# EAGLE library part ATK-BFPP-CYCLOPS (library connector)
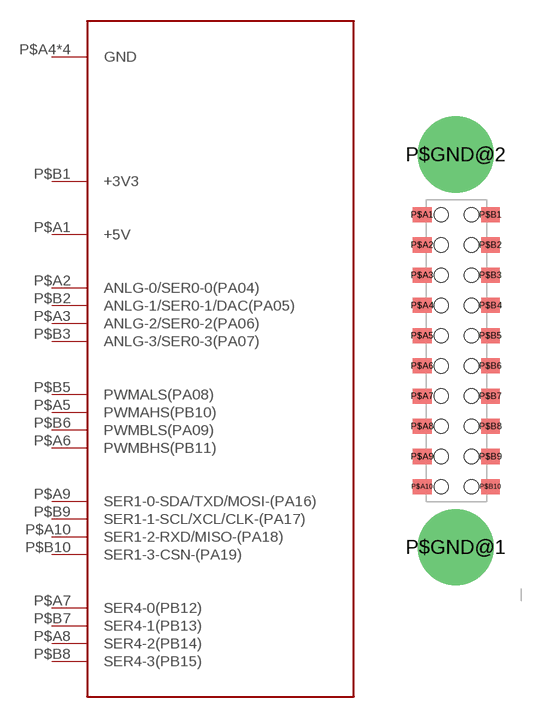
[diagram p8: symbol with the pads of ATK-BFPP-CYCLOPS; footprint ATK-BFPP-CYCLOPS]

Designator prefix J

## ATK-BFPP-CYCLOPSCYCLOPS  [ATK-BFPP-CYCLOPS]
P$A1  +5V
P$A2  ANLG-0/SER0-0(PA04)
P$A3  ANLG-2/SER0-2(PA06)
P$A4  GND
P$A5  PWMAHS(PB10)
P$A6  PWMBHS(PB11)
P$A7  SER4-0(PB12)
P$A8  SER4-2(PB14)
P$A9  SER1-0-SDA/TXD/MOSI-(PA16)
P$A10  SER1-2-RXD/MISO-(PA18)
P$B1  +3V3
P$B2  ANLG-1/SER0-1/DAC(PA05)
P$B3  ANLG-3/SER0-3(PA07)
P$B4  GND
P$B5  PWMALS(PA08)
P$B6  PWMBLS(PA09)
P$B7  SER4-1(PB13)
P$B8  SER4-3(PB15)
P$B9  SER1-1-SCL/XCL/CLK-(PA17)
P$B10  SER1-3-CSN-(PA19)
P$GND@1  GND
P$GND@2  GND

## Footprint ATK-BFPP-CYCLOPS (pad centres in mm)
smd 1.57 x 1.27: P$A1 -2.815,11.43; P$A2 -2.815,8.89; P$A3 -2.815,6.35; P$A4 -2.815,3.81; P$A5 -2.815,1.27; P$A6 -2.815,-1.27; P$A7 -2.815,-3.81; P$A8 -2.815,-6.35; P$A9 -2.815,-8.89; P$A10 -2.815,-11.43; P$B1 2.925,11.43; P$B2 2.925,8.89; P$B3 2.925,6.35; P$B4 2.925,3.81; P$B5 2.925,1.27; P$B6 2.925,-1.27; P$B7 2.925,-3.81; P$B8 2.925,-6.35; P$B9 2.925,-8.89; P$B10 2.925,-11.43
drill 4.4 pad 6.4: P$GND@1 0,-16.5; P$GND@2 0,16.5
hole 1.2 at -1.215,11.43
hole 1.2 at -1.215,8.89
hole 1.2 at -1.215,6.35
hole 1.2 at -1.215,3.81
hole 1.2 at -1.215,1.27
hole 1.2 at -1.215,-1.27
hole 1.2 at -1.215,-3.81
hole 1.2 at -1.215,-6.35
hole 1.2 at -1.215,-8.89
hole 1.2 at -1.215,-11.43
hole 1.2 at 1.325,11.43
hole 1.2 at 1.325,8.89
hole 1.2 at 1.325,6.35
hole 1.2 at 1.325,3.81
hole 1.2 at 1.325,1.27
hole 1.2 at 1.325,-1.27
hole 1.2 at 1.325,-3.81
hole 1.2 at 1.325,-6.35
hole 1.2 at 1.325,-8.89
hole 1.2 at 1.325,-11.43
